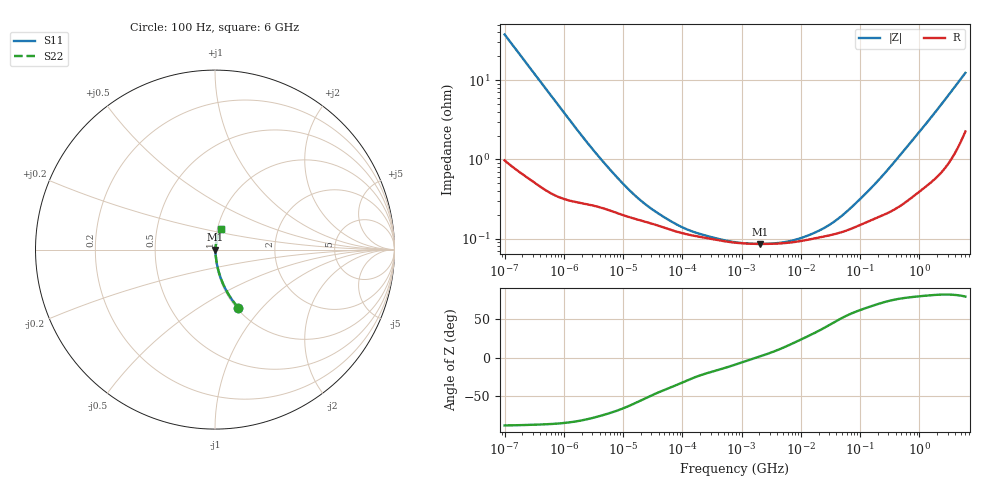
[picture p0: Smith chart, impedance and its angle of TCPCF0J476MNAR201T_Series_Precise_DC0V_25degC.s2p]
! TCPCF0J476MNAR201T Polymer Tantalum Capacitor Sparameter Model
! Model Generated by Samsung Electro-Mechanics
! Samsung Sparameter Version 5.0
! Date : Oct-10-2024
! Products : Polymer Tantalum Capacitor
! Characteristics :
!  Nominal Capacitance = 47uF
!  Capacitance Tolerance = +/-20%
!  ESR = 200 mohm max at 100kHz
!  Rated Voltage = 6.3Vdc
!  Size = 0805(unit:inch), 2012(unit:mm)
!  Length = 2.00+/-0.20mm
!  Width = 1.25+/-0.20mm
!  Thickness = 0.80+/-0.10mm
!  Lineup = Conductive Polymer Type
!  Feature = PCF
!  Measurement Temperature : 25degC.
!  DC bias Value = 0V
!  Frequency : 100Hz ~ 6GHz
! External Node Assignments :
!  1  o---||---o  2
# MHz S RI R 50.0
! Freq.  Real(S11)  Im(S11)  Real(S12)  Im(S12)  Real(S21)  Im(S21)  Real(S22)  Im(S22)
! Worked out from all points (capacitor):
!   300 points, 100 Hz to 6 GHz, reference 50 ohm
!   read as one part in series: C = 42.1 uF near 106.2 Hz
!   lowest |Z| = 86.2 mohm at 2.081 MHz (marker M1)
!   series resonance near 1.801 MHz, so ESL is about 190 pH
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0.0001  0.1306 -0.3243  0.8694 0.3243  0.8694 0.3243  0.1306 -0.3243
0.0001714451  0.0528 -0.2081  0.9472 0.2081  0.9472 0.2081  0.0528 -0.2081
0.0003517965  0.0164 -0.1068  0.9836 0.1068  0.9836 0.1068  0.0164 -0.1068
0.0007664292  0.00596 -0.0502  0.994 0.0502  0.994 0.0502  0.00596 -0.0502
0.001998454  0.00319 -0.0197  0.9968 0.0197  0.9968 0.0197  0.00319 -0.0197
0.004907976  0.00245 -0.0085  0.9975 0.0085  0.9975 0.0085  0.00245 -0.0085
0.01135264  0.00194 -0.00403  0.9981 0.00403  0.9981 0.00403  0.00194 -0.00403
0.02066501  0.00169 -0.00243  0.9983 0.00243  0.9983 0.00243  0.00169 -0.00243
0.03993819  0.00146 -0.00147  0.9985 0.00147  0.9985 0.00147  0.00146 -0.00147
0.08195114  0.00122 -0.000869  0.9988 0.000869  0.9988 0.000869  0.00122 -0.000869
0.1405012  0.00111 -0.000581  0.9989 0.000581  0.9989 0.000581  0.00111 -0.000581
0.3450549  0.000979 -0.000311  0.999 0.000311  0.999 0.000311  0.000979 -0.000311
0.7981464  0.000891 -0.000141  0.9991 0.000141  0.9991 0.000141  0.000891 -0.000141
2.081156  0.000861 2.43e-05  0.9991 -2.43e-05  0.9991 -2.43e-05  0.000861 2.43e-05
6.117227  0.00089 0.00025  0.9991 -0.00025  0.9991 -0.00025  0.00089 0.00025
15.95059  0.001 0.000598  0.999 -0.000598  0.999 -0.000598  0.001 0.000598
29.03458  0.0011 0.000971  0.9989 -0.000971  0.9989 -0.000971  0.0011 0.000971
52.85115  0.00124 0.00162  0.9988 -0.00162  0.9988 -0.00162  0.00124 0.00162
137.8087  0.00167 0.00365  0.9983 -0.00365  0.9983 -0.00365  0.00167 0.00365
318.7652  0.00223 0.00763  0.9978 -0.00763  0.9978 -0.00763  0.00223 0.00763
1922.593  0.00743 0.0398  0.9926 -0.0398  0.9926 -0.0398  0.00743 0.0398
6000  0.0357 0.1145  0.9643 -0.1145  0.9643 -0.1145  0.0357 0.1145
